PROGRAM PRG_Recipe			(*只做参数保存*)
VAR
	fbRecipe			: FB_Recipe;
	eFileType			: E_FileType :=eFileType_BIN;
END_VAR

;
fbRecipe(
	bRunOnCeDevice		:= FALSE,					(* TRUE--CE系统, FALSE--非CE系统*)
	sgFilePath			:= '\Data\Recipe\',			(* 文件路径, 默认是 \Data\Recipe\' *)
	eFileType			:= eFileType,				(* 文件类型, 默认是XML, 只支持 eFileType_XML 和 eFileType_BIN 两种类型 *)
	pRecData			:= ADR(sRecData),			(* 配方参数首地址 *)
	pBakData			:= ADR(_sRecData),			(* 配方备份的首地址, 保存上一次的参数值, 用来比较参数是否有变化 *)
	nRecSize			:= SIZEOF(sRecData),		(* 配方总字节数 *)
	tAutoSaveRec		:= T#3S,					(* 参数变化后, 延时保存(写文件) *)
	bInitialDone		=> ,						(* 初始化完成 *)
	bDone				=> ,						(* 读写完成 *)
	bBusy				=> ,						(* 读写中 *)
	bError				=> ,						(* 读写失败 *)
	nErrorId			=> );						(* 错误代码 *)

END_PROGRAM
